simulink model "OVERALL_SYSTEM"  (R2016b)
settings: Solver=VariableStepAuto  StartTime=0.0  StopTime=12  FixedStep=0.1e-3  RelTol=1e-3
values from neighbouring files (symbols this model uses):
  beta_max = 90    [SYSTEM_PATAMETERS.m]
  beta_min = 0    [SYSTEM_PATAMETERS.m]
  beta_r = 4    [SYSTEM_PATAMETERS.m]
  c1 = 0.5    [SYSTEM_PATAMETERS.m]
  c2 = 116    [SYSTEM_PATAMETERS.m]
  c3 = 0.4    [SYSTEM_PATAMETERS.m]
  c4 = 5    [SYSTEM_PATAMETERS.m]
  c5 = 21    [SYSTEM_PATAMETERS.m]
  c6 = 0    [SYSTEM_PATAMETERS.m]
  Cdc = 0.08    [SYSTEM_PATAMETERS.m]
  Cp_max = 0.41    [SYSTEM_PATAMETERS.m]
  fn = 50    [SYSTEM_PATAMETERS.m]
  I2base = (2*Sn)/(3*V2base)    [SYSTEM_PATAMETERS.m]
  Ibase = (2*Sn)/(3*Vbase)    [SYSTEM_PATAMETERS.m]
  Idcbase = ((3/2)*Vbase*Ibase)/Vdcbase    [SYSTEM_PATAMETERS.m]
  J = Sn*2*H/(wm^2)    (= 133997.265367)    [SYSTEM_PATAMETERS.m]
  Ki = Kp/Ti    (= 750)    [SYSTEM_PATAMETERS.m]
  Ki_SSC = Kp_SSC/Ti_SSC    [SYSTEM_PATAMETERS.m]
  Kib = Kpb/Tb    (= 25)    [SYSTEM_PATAMETERS.m]
  Kibv = Kpbv/Tibv    [SYSTEM_PATAMETERS.m]
  Kidc = Kpdc/Tidc    [SYSTEM_PATAMETERS.m]
  Kiq = Kpq/Tiq    [SYSTEM_PATAMETERS.m]
  Kiw = Kpw/Tiw    (= 1)    [SYSTEM_PATAMETERS.m]
  Kp = xs_filter/(2*wbase*Ta)    (= 12.7323954474)    [SYSTEM_PATAMETERS.m]
  Kp_SSC = ls_filter/(2*wbase*Te)    [SYSTEM_PATAMETERS.m]
  Kpb = 5    [SYSTEM_PATAMETERS.m]
  Kpbv = ls_filterb/(2*wbase*Te)    [SYSTEM_PATAMETERS.m]
  Kpdc = (Vdcbase*Tc)/(V2*a*Teq)    [SYSTEM_PATAMETERS.m]
  Kpq = Tf_Q_const*rs_filter/(a*Teq)    [SYSTEM_PATAMETERS.m]
  Kpw = 4    [SYSTEM_PATAMETERS.m]
  lambda_opt = 7.95    [SYSTEM_PATAMETERS.m]
  ls = Ls/Lbase    [SYSTEM_PATAMETERS.m]
  ls_filter = Ls_filter/Lbase    [SYSTEM_PATAMETERS.m]
  Ls_filter = Xs_filter/we    [SYSTEM_PATAMETERS.m]
  polepairs = poles/2    (= 115)    [SYSTEM_PATAMETERS.m]
  psim_pu = psim/psibase    [SYSTEM_PATAMETERS.m]
  r = 26    [SYSTEM_PATAMETERS.m]
  rho = 1.225    [SYSTEM_PATAMETERS.m]
  Rs = rs*Zbase    [SYSTEM_PATAMETERS.m]
  Rs_filter = rs_filter*Zbase    [SYSTEM_PATAMETERS.m]
  Sn = 250e3    (= 250000)    [SYSTEM_PATAMETERS.m]
  Ta = Tsw/2    (= 0.0001)    [SYSTEM_PATAMETERS.m]
  Ts = 1e-5    (= 1e-05)    [SYSTEM_PATAMETERS.m]
  V2 = 400    [SYSTEM_PATAMETERS.m]
  V2base = V2*sqrt(2)/sqrt(3)    [SYSTEM_PATAMETERS.m]
  Vbase = V1*sqrt(2)/sqrt(3)    [SYSTEM_PATAMETERS.m]
  Vdcbase = 3*Vbase    [SYSTEM_PATAMETERS.m]
  w2base = 2*pi*fn    (= 314.159265359)    [SYSTEM_PATAMETERS.m]
  wbase = 2*pi*fn    (= 314.159265359)    [SYSTEM_PATAMETERS.m]
  wm = nm*pi/30    (= 2.73181969877)    [SYSTEM_PATAMETERS.m]
undefined symbols (not defined in the file or in its folder): bridge, by, dend, DiscIntNeverNeededParam, established, Flux, h, Ion, K, Ld, linkage, Lithium, Lq, magnets, numd, phase, Pm0, pulses, sigbuilder_block, Td, Three, Tlim, Tr, V
libraries: powerlib x32, powerlib_meascontrol x14, simulink x10, powerlib_extras x2, sps_avr x1, electricdrivelib x1
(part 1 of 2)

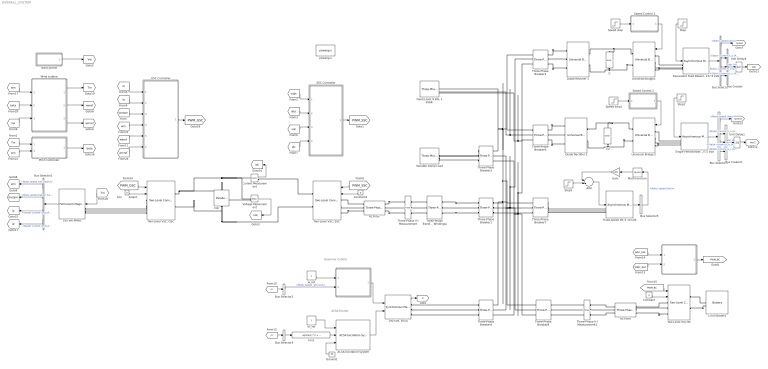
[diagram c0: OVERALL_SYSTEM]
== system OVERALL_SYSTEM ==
  note: Governor Control
  note: AC5A Exciter
  " " : Subsystem
  " " : Subsystem
  "140 kVA, EESG" : powerlib/Machines/Synchronous Machine pu Fundamental  PresetModel=No  MechanicalLoad=Mechanical power Pm  ShowDetailedParameters=on  RotorType=Round  Units=per unit fundamental parameters  MeasurementBus=off  NominalParameters="[ 140e3 V2   fn]"  Stator="[ 0.0317  0.114  1.19  0.36 ]"  Field="[ 5.79E-04  0.114]"  Dampers2=[0.0652, 0.5134, 0.0287, 0.2553, 7.765e-3, 0.9167 ]  Dampers1="[ 1.17E-02  0.182  1.97E-02  0.384 ]"  Mechanical=[ 0.7 0 20]  PolePairs=2  InitialConditions="[ 0  36.87  0  0  0  0  0 0  1 ]"  SetSaturation=off  Saturation=[0.6404,0.7127,0.8441,0.9214,0.9956,1.082,1.19,1.316,1.457;0.7,0.7698,0.8872,0.9466,0.9969,1.046,1.1,1.151,1.201]  LoadFlowParameters=[1,0,0,0,0]  TsPowergui=0  TsBlock=-1  IterativeModel=Trapezoidal non iterative  IterativeDiscreteModel=Trapezoidal non iterative  BusType=PV  Pref=0  Qref=0  Qmin=-inf  Qmax=inf  PLF=0  QLF=0
  250 kW PMSG : powerlib/Machines/Permanent Magnet Synchronous Machine  NbPhases=3  FluxDistribution=Sinusoidal  RotorType=Round  MechanicalLoad=Torque Tm  PresetModel=No  ShowDetailedParameters=on  MeasurementBus=off  Resistance=Rs  Inductance=8.5e-3  dqInductances=[Ld, Lq]  La=Ls  MachineConstant=Flux linkage established by magnets (V.s)  Flux=1.5  VoltageCst=31288.039  TorqueCst=258.75  Flat=120  Mechanical=[J 0 polepairs 0]  PolePairs=273  InitialConditions=[1.76,15, 0,0]  InitialConditions5ph=[0 0 0 0 0 0]  TsPowergui=0  TsBlock=Ts  RefAngle=Aligned with phase A axis (original Park)
  AC5A Excitation System : sps_avr/AC5A Excitation System  Tr=20e-3  KaTa=[500 0.02]  VRminmax=[-7.3 7.3]  KfTf=[0.03 1 0 0]  KeTe=[1 0.02]  Efd12=[5.6 0.75*5.6]  SeEfd12=[0.86 0.5]  v0=[1 1]  TsBlock=0
  Add : Sum
  Bus Creator : BusCreator  Inputs=3
  Bus Creator1 : BusCreator  Inputs=3
  Bus Selector : BusSelector  OutputSignals=Mechanical.Rotor speed (wm),Stator measurements.Stator current is_a (A),Stator measurements.Stator current is_b (A),Stator measurements.Stator current is_c (A)
  Bus Selector1 : BusSelector  OutputSignals=Rotor speed wm (rad/s),Rotor angle thetam (rad),Stator current is_q (A),Stator current is_d (A)
  Bus Selector2 : BusSelector  OutputSignals="Mechanical.Rotor speed  wm (pu)"
  Bus Selector3 : BusSelector  OutputSignals="dq0 components.Stator voltage  vq (pu),dq0 components.Stator voltage  vd (pu)"  OutputAsBus=on
  Bus Selector4 : BusSelector  OutputSignals=Mechanical.Rotor speed (wm),Stator measurements.Stator current is_a (A),Stator measurements.Stator current is_b (A),Stator measurements.Stator current is_c (A)
  Bus Selector5 : BusSelector  OutputSignals=Mechanical.Rotor speed (wm)
  C : powerlib/Elements/Series RLC Branch  LConnTagsString=__new0  RConnTagsString=__new0  BranchType=C  Resistance=1  Inductance=1e-3  SetiL0=off  InitialCurrent=0  Capacitance=7.5e-3  Setx0=on  InitialVoltage=sqrt(2)*400  Measurements=None
  C2 : powerlib/Elements/Series RLC Branch  LConnTagsString=__new0  RConnTagsString=__new0  BranchType=C  Resistance=1  Inductance=1e-3  SetiL0=off  InitialCurrent=0  Capacitance=7.5e-3  Setx0=on  InitialVoltage=sqrt(2)*400  Measurements=None
  Cdc : powerlib/Elements/Parallel RLC Branch  LConnTagsString=a  RConnTagsString=__new0  BranchType=C  Resistance=1e12  Inductance=1e-3  SetiL0=off  InitialCurrent=0  Capacitance=Cdc  Setx0=on  InitialVoltage=Vdcbase  Measurements=None
  Con        2stant : Constant  Value=0
  Constant : Constant  Value=0
  Constant1 : Constant  Value=0
  Current Measurement : powerlib/Measurements/Current Measurement  PhasorSimulation=off  OutputType=Complex  PSBequivalent=0
  Diode Rectifier 1 : powerlib/Power Electronics/Universal Bridge  Arms=3  SnubberResistance=1e5  SnubberCapacitance=inf  Device=Diodes  Ron=1e-3  Lon=0  ForwardVoltages="[  0  0  ]"  ForwardVoltage=0  GTOparameters=[ 10e-6 , 20e-6 ]  IGBTparameters=[ 1e-6 , 2e-6 ]  Measurements=None  Measurements_2=None  converterType=Rectifier
  Diode Rectifier 2 : powerlib/Power Electronics/Universal Bridge  Arms=3  SnubberResistance=1e5  SnubberCapacitance=inf  Device=Diodes  Ron=1e-3  Lon=0  ForwardVoltages="[  0  0  ]"  ForwardVoltage=0  GTOparameters=[ 10e-6 , 20e-6 ]  IGBTparameters=[ 1e-6 , 2e-6 ]  Measurements=None  Measurements_2=None  converterType=Rectifier
  "Equivalent Feed Blower, 137.5 kVA" : powerlib/Machines/Asynchronous Machine SI Units  RotorType=Squirrel-cage  PresetModel=No  MechanicalLoad=Torque Tm  ShowDetailedParameters=on  ReferenceFrame=Stationary  Units=SI  MeasurementBus=off  NominalParameters=[137.5e3 400 50]  Stator=[ 0.087 0.8e-3 ]  Rotor="[ 0.228  0.8e-3 ]"  Cage1=[0.4155 0.002066]  Cage2=[0.4168 0.0003495]  Lm=0.0354  Mechanical="[1.662  0.01 2 ]"  PolePairs=2  InitialConditions=[1 0 0 0 0 0 0 0]  SimulateSaturation=off  Saturation=[14.03593122, 27.81365428, 53.79336849, 72.68890987, 97.98006896, 148.6815601, 215.7428561, 302.9841135, 428.7778367 ; 230, 322, 414, 460, 506, 552, 598, 644, 690]  LoadFlowParameters=1492000  TsPowergui=0  TsBlock=-1  IterativeModel=Trapezoidal non iterative  IterativeDiscreteModel=Trapezoidal non iterative  Pmec=72.6e3
  Fcn1 : Fcn  Expr=sqrt(u(1)^2 + u(2)^2)
  "Fixed Load, 9 kW, 1 kVAR " : powerlib/Elements/Three-Phase Series RLC Load  LConnTagsString=A|B|C  Configuration=Y (grounded)  NominalVoltage=400  Vabc=[1e3 1e3 1e3]  Vabcp=[1e3 1e3 1e3]  NominalFrequency=50  UnbalancedPower=off  ActivePower=2e3  InductivePower=0.5e3  CapacitivePower=0  Pabc=[10e3 9e3 11e3]  QLabc=[100 90 110]  QCabc=[100 90 110]  Pabcp=[10e3 9e3 11e3]  QLabcp=[100 90 110]  QCabcp=[100 90 110]  Measurements=None  LoadType=constant Z
  "Fixed-speed IM, 5-10 kVA" : powerlib/Machines/Asynchronous Machine pu Units  RotorType=Squirrel-cage  PresetModel=No  MechanicalLoad=Torque Tm  ShowDetailedParameters=on  ReferenceFrame=Rotor  Units=pu  MeasurementBus=off  NominalParameters=[10000 400 50]  Stator=[0.01965 0.0397]  Rotor=[0.01909 0.0397]  Cage1=[0.01909 0.0397]  Cage2=[0.01909 0.0397]  Lm=1.354  Mechanical=[0.6 0.05479 2]  PolePairs=2  InitialConditions="[ 1,0   0,0,0   0,0,0 ]"  SimulateSaturation=off  Saturation="[0.212,0.4201,0.8125,1.0979,1.4799,2.2457,3.2586,4.5763,6.4763 ;   0.5,0.7,0.9,1,1.1,1.2 ,1.3,1.4,1.5]"  LoadFlowParameters=0  TsPowergui=0  TsBlock=-1  IterativeModel=Trapezoidal non iterative  IterativeDiscreteModel=Trapezoidal non iterative  Pmec=0
  GSC Controller : Subsystem
  Gain : Gain  Gain=0.85
  Ground1 : Ground
  Li-ion Battery : electricdrivelib/Extra Sources/Battery  BatType=Lithium-Ion  ShowTempParam=off  ThermalPreset=no  NomV=Vb  NomQ=Ahb  SOC=SOC0  Batt_Tr=0.1  PresetModel=on  MaxQ=100  MinV=739.5  FullV=1147.6913  Dis_rate=43.4783  R=0.0986  Normal_OP=90.4348  expZone="[1065.2605      4.9130435]"  current=[50]  Units=Ampere-hour  Tci=20  NomT=25  T2=0  MaxQ2=2.208  FullV2=3.45  Normal_OP2=2.8  expZone2="[3.22        0.23]"  Rca=0.6  ti=1000  Dp=0
  Math Function : Math  Operator=square
  Pitch Controller : Subsystem
  RL Filter : powerlib/Elements/Three-Phase Series RLC Branch  LConnTagsString=A|B|C  RConnTagsString=A|B|C  BranchType=RL  Resistance=Rs_filter  Inductance=Ls_filter  Capacitance=1e-6  Measurements=None
  RL-Filter : powerlib/Elements/Three-Phase Series RLC Branch  LConnTagsString=A|B|C  RConnTagsString=A|B|C  BranchType=RL  Resistance=Rs_filter  Inductance=Ls_filter  Capacitance=1e-6  Measurements=None
  SSC Controller : Subsystem
  "Single Feed Blower, 27.5 kVA" : powerlib/Machines/Asynchronous Machine SI Units  RotorType=Squirrel-cage  PresetModel=No  MechanicalLoad=Torque Tm  ShowDetailedParameters=on  ReferenceFrame=Stationary  Units=SI  MeasurementBus=off  NominalParameters=[27.5e3 400 50]  Stator=[ 0.087 0.8e-3 ]  Rotor="[ 0.228  0.8e-3 ]"  Cage1=[0.4155 0.002066]  Cage2=[0.4168 0.0003495]  Lm=0.0354  Mechanical="[1.662  0.01 2 ]"  PolePairs=2  InitialConditions=[1 0 0 0 0 0 0 0]  SimulateSaturation=off  Saturation=[14.03593122, 27.81365428, 53.79336849, 72.68890987, 97.98006896, 148.6815601, 215.7428561, 302.9841135, 428.7778367 ; 230, 322, 414, 460, 506, 552, 598, 644, 690]  LoadFlowParameters=1492000  TsPowergui=0  TsBlock=-1  IterativeModel=Trapezoidal non iterative  IterativeDiscreteModel=Trapezoidal non iterative  Pmec=72.6e3
  Speed step : Step  Time=3  After=150  SampleTime=0
  Speed step1 : Step  Time=3  After=150  SampleTime=0
  Speed Control 1 : Subsystem
  Speed Control 2 : Subsystem
  Step : Step  Time=4  After=240  SampleTime=0
  Step1 : Step  Time=4  After=150  SampleTime=0
  Step2 : Step  Time=6  After=0.15  SampleTime=0
  Three-Phase Transformer (Two Windings) : powerlib/Elements/Three-Phase Transformer (Two Windings)  Winding1Connection=Yg  Winding2Connection=Yg  CoreType=Three single-phase transformers  SetSaturation=off  Hysteresis=off  DataFile='hysteresis'  SetInitialFlux=off  Measurements=None  UNITS=pu  NominalPower=[ 250e3 , 50 ]  Winding1=[ 690 , 0.002 , 0.08 ]  Winding2=[ 400 , 0.002 , 0.08 ]  Rm=500  Lm=500  L0=0.5  Saturation=[ 0,0 ; 0.0024,1.2 ; 1.0,1.52 ]  InitialFluxes=[ 0.8 , -0.8 , 0.7 ]  MoreParameters=off  BreakLoop=off  DataType=off  TransfoNumber=1
  Three-Phase V-I Measurement : powerlib/Measurements/Three-Phase V-I Measurement  VoltageMeasurement=phase-to-phase  SetLabelV=on  LabelV=vabc  Vpu=off  VpuLL=off  CurrentMeasurement=yes  SetLabelI=on  LabelI=iabc  Ipu=off  Pbase=6e6  Vbase=690  OutputType=Complex  PhasorSimulation=off  PSBequivalent=0
  Three-Phase V-I Measurement1 : powerlib/Measurements/Three-Phase V-I Measurement  VoltageMeasurement=phase-to-phase  SetLabelV=on  LabelV=Vabc_bat  Vpu=off  VpuLL=off  CurrentMeasurement=yes  SetLabelI=on  LabelI=Iabc_bat  Ipu=off  Pbase=6e6  Vbase=690  OutputType=Complex  PhasorSimulation=off  PSBequivalent=0
  Three-Phase Breaker{1..3,6} (4 alike) : powerlib/Elements/Three-Phase Breaker  InitialState=open  SwitchA=on  SwitchB=on  SwitchC=on  SwitchTimes=2.9  External=off  BreakerResistance=0.01  SnubberResistance=1e6  SnubberCapacitance=inf  Measurements=None
  Three-Phase Breaker4 : powerlib/Elements/Three-Phase Breaker  InitialState=open  SwitchA=on  SwitchB=on  SwitchC=on  SwitchTimes=5.25  External=off  BreakerResistance=0.01  SnubberResistance=1e6  SnubberCapacitance=inf  Measurements=None
  Three-Phase Breaker7 : powerlib/Elements/Three-Phase Breaker  InitialState=open  SwitchA=on  SwitchB=on  SwitchC=on  SwitchTimes=6  External=off  BreakerResistance=0.01  SnubberResistance=1e6  SnubberCapacitance=inf  Measurements=None
  Three-Phase Breaker8 : powerlib/Elements/Three-Phase Breaker  InitialState=open  SwitchA=on  SwitchB=on  SwitchC=on  SwitchTimes=5.25  External=off  BreakerResistance=0.01  SnubberResistance=1e6  SnubberCapacitance=inf  Measurements=None
  Two-Level VSC BC : powerlib/Power Electronics/Two-Level Converter  ModelType=Switching devices  Ron=1e-3  Rs=1e6  Cs=inf  Vforward=[0,0]  Ron_Diode=1e-3  Rs_Diode=1e6  Cs_Diode=inf  Vf_Diode=1e-3  Rs_CurrentSource=inf
  "Two-Level VSC, GSC" : powerlib/Power Electronics/Two-Level Converter  ModelType=Switching devices  Ron=1e-3  Rs=1e6  Cs=inf  Vforward=[0,0]  Ron_Diode=1e-3  Rs_Diode=1e6  Cs_Diode=inf  Vf_Diode=1e-3  Rs_CurrentSource=inf
  "Two-Level VSC, SSC" : powerlib/Power Electronics/Two-Level Converter  ModelType=Switching devices  Ron=1e-3  Rs=1e6  Cs=inf  Vforward=[0,0]  Ron_Diode=1e-3  Rs_Diode=1e6  Cs_Diode=inf  Vf_Diode=1e-3  Rs_CurrentSource=inf
  Unit Delay1 : UnitDelay  SampleTime=Ts
  Unit Delay4 : UnitDelay  SampleTime=Ts
  Universal Bridge 2 : powerlib/Power Electronics/Universal Bridge  Arms=3  SnubberResistance=1e5  SnubberCapacitance=inf  Device=IGBT / Diodes  Ron=1e-3  Lon=0  ForwardVoltages="[  0  0  ]"  ForwardVoltage=0  GTOparameters=[ 10e-6 , 20e-6 ]  IGBTparameters=[ 1e-6 , 2e-6 ]  Measurements=None  Measurements_2=None  converterType=Rectifier
  Universal Bridge1 : powerlib/Power Electronics/Universal Bridge  Arms=3  SnubberResistance=1e5  SnubberCapacitance=inf  Device=IGBT / Diodes  Ron=1e-3  Lon=0  ForwardVoltages="[  0  0  ]"  ForwardVoltage=0  GTOparameters=[ 10e-6 , 20e-6 ]  IGBTparameters=[ 1e-6 , 2e-6 ]  Measurements=None  Measurements_2=None  converterType=Rectifier
  Variable Dump Load : powerlib/Elements/Three-Phase Series RLC Load  LConnTagsString=A|B|C  Configuration=Y (grounded)  NominalVoltage=400  Vabc=[1e3 1e3 1e3]  Vabcp=[1e3 1e3 1e3]  NominalFrequency=50  UnbalancedPower=off  ActivePower=10e3  InductivePower=1e3  CapacitivePower=0  Pabc=[10e3 9e3 11e3]  QLabc=[100 90 110]  QCabc=[100 90 110]  Pabcp=[10e3 9e3 11e3]  QLabcp=[100 90 110]  QCabcp=[100 90 110]  Measurements=None  LoadType=constant Z
  Voltage Measurement : powerlib/Measurements/Voltage Measurement  PhasorSimulation=off  OutputType=Complex  PSBequivalent=0
  Vt_ref : Constant
  Wind profile : Subsystem  Tag=STV Subsys  LoadFcn=sigbuilder_block('load');  StartFcn=sigbuilder_block('start');  StopFcn=sigbuilder_block('stop');  ClipboardFcn=sigbuilder_block('clipboard');
  Wind turbine : Subsystem
  powergui : powerlib/powergui  Priority=1  SimulationMode=Discrete  SolverType=Tustin/Backward Euler (TBE)  SampleTime=Ts  frequency=60  SPID=off  DisableSnubberDevices=off  DisableRonSwitches=off  DisableVfSwitches=off  SwTol=0  DisplayEquations=off  Interpol=off  ExternalGateDelay=off  methode=off  Ts=10  FunctionMessages=off  echomessages=off  HookPort=off  EnableUseOfTLC=off  x0status=blocks  frequencyindice=50  Pbase=100e6  ErrMax=1e-4  Iterations=50  UnitsV=kV  UnitsW=MW  buscounter=0  RestoreLinks=warning  ResistiveCurrentMeasurement=off  Frange=[0:2:500]  Ylog=off  Xlog=on  ShowGrid=off  save=off  variable=ZData  structure=0  ZoomFFT=off  StartTime=0.0  cycles=1  DisplayStyle=1  fundamental=60  FreqAxis=off  MaxFrequency=1000  frequencyindicesteady=1  RmsSteady=1  display=off
  w_ref : Constant
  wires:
  Bus Selector1/2 -> [thetam]  "<Rotor angle thetam (rad)>"
  Bus Selector1/1 -> [wm]  "<Rotor speed wm (rad/s)>"
  Bus Selector1/3 -> [iq]  "<Stator current is_q (A)>"
  Bus Selector1/4 -> [id]  "<Stator current is_d (A)>"
  Con        2stant/1 -> "Two-Level VSC, GSC"/2
  [Tm] -> 250 kW PMSG/1
  [beta] -> Wind turbine/2(Beta [deg])
  [wm] -> Wind turbine/1("wm [rad/s] ")
  Wind turbine/1(Tm [Nm]) -> [Tm]
  Wind turbine/2(we_ref [pu]) -> [weref]
  [PWM_GSC] -> "Two-Level VSC, GSC"/1
  GSC Controller/1(Uref) -> [PWM_GSC]
  [id] -> GSC Controller/1(Id [A])
  [iq] -> GSC Controller/2(Iq [A])
  [thetam] -> GSC Controller/3(Thetam [rad])
  [wm] -> GSC Controller/4(Wm [rad/s])
  [weref] -> GSC Controller/5(We_ref [pu])
  Constant1/1 -> "Two-Level VSC, SSC"/2
  [PWM_SSC] -> "Two-Level VSC, SSC"/1
  Voltage Measurement/1 -> [vdc]
  Current Measurement/1 -> [idc]
  SSC Controller/1(Uref) -> [PWM_SSC]
  [vabc] -> SSC Controller/1(vabc [V])
  [iabc] -> SSC Controller/2(iabc [A])
  [vdc] -> SSC Controller/3(vdc [V])
  [idc] -> SSC Controller/4(idc [A])
  [Tm] -> Pitch Controller/1(Tm [Nm])
  Pitch Controller/1(Beta [deg]) -> [beta]
  [Vw] -> Wind turbine/3(V_wind [m/s])
  [wm] -> Pitch Controller/2(wm [rad/s])
  Wind turbine/3(wm_ref [pu]) -> [wmref]
  [wmref] -> GSC Controller/6(Wm_ref [pu])
  250 kW PMSG/1 -> Bus Selector1/1
  Wind profile/1(Final Wind) -> [Vw]
  Ground1/1 -> AC5A Excitation System/3
  AC5A Excitation System/1 -> "140 kVA, EESG"/2
  Vt_ref/1 -> AC5A Excitation System/1
  Fcn1/1 -> AC5A Excitation System/2
  Bus Selector3/1 -> Fcn1/1
  Bus Selector2/1 -> " "/2(w (pu))  "<Rotor speed  wm (pu)>"
  w_ref/1 -> " "/1(wref (pu))
  " "/1(Pmec (pu)) -> "140 kVA, EESG"/1
  "140 kVA, EESG"/1 -> [m]
  [m] -> Bus Selector2/1
  [m] -> Bus Selector3/1
  Constant/1 -> Two-Level VSC BC/2
  " "/1(Vref) -> [PWM_BC]
  [Vabc_bat] -> " "/2(Vabc [V])
  [Iabc_bat] -> " "/1(Iabc [A])
  [PWM_BC] -> Two-Level VSC BC/1
  Unit Delay4/1 -> [Iabc]
  Bus Selector/3 -> Bus Creator/2  "<Stator current is_b (A)>"
  Bus Creator/1 -> Unit Delay4/1  "Iabc (A)"
  Bus Selector/2 -> Bus Creator/1  "<Stator current is_a (A)>"
  Bus Selector/4 -> Bus Creator/3  "<Stator current is_c (A)>"
  Speed Control 1/1(pulses) -> Universal Bridge1/1
  Step/1 -> "Equivalent Feed Blower, 137.5 kVA"/1
  Speed step/1 -> Speed Control 1/1(speed)
  "Equivalent Feed Blower, 137.5 kVA"/1 -> Bus Selector/1
  Bus Selector/1 -> [Speed]  "<Rotor speed (wm)>"
  Speed Control 2/1(pulses) -> Universal Bridge 2/1
  Step1/1 -> "Single Feed Blower, 27.5 kVA"/1
  Speed step1/1 -> Speed Control 2/1(speed)
  Unit Delay1/1 -> [Iabc2]
  Bus Selector4/3 -> Bus Creator1/2  "<Stator current is_b (A)>"
  Bus Creator1/1 -> Unit Delay1/1  "Iabc (A)"
  Bus Selector4/2 -> Bus Creator1/1  "<Stator current is_a (A)>"
  Bus Selector4/4 -> Bus Creator1/3  "<Stator current is_c (A)>"
  "Single Feed Blower, 27.5 kVA"/1 -> Bus Selector4/1
  Bus Selector4/1 -> [Speed2]  "<Rotor speed (wm)>"
  Step2/1 -> Add/2
  "Fixed-speed IM, 5-10 kVA"/1 -> Bus Selector5/1
  Bus Selector5/1 -> Math Function/1  "<Rotor speed (wm)>"
  Add/1 -> "Fixed-speed IM, 5-10 kVA"/1
  Math Function/1 -> Gain/1
  Gain/1 -> Add/1
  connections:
  Three-Phase Breaker3/RConn1 -- Variable Dump Load/LConn1
  Variable Dump Load/LConn2 -- Three-Phase Breaker3/RConn2
  Three-Phase Breaker3/RConn3 -- Variable Dump Load/LConn3
  "140 kVA, EESG"/RConn1 -- Three-Phase Breaker4/LConn1
  "140 kVA, EESG"/RConn2 -- Three-Phase Breaker4/LConn2
  "140 kVA, EESG"/RConn3 -- Three-Phase Breaker4/LConn3
  Cdc/RConn1 -- "Two-Level VSC, SSC"/RConn2 -- Voltage Measurement/LConn2 -- "Two-Level VSC, GSC"/RConn2
  "Two-Level VSC, GSC"/RConn1 -- Current Measurement/LConn1 -- Voltage Measurement/LConn1 -- Cdc/LConn1
  "Two-Level VSC, SSC"/RConn1 -- Current Measurement/RConn1
  RL Filter/LConn3 -- Three-Phase V-I Measurement/RConn3
  "Two-Level VSC, SSC"/LConn1 -- RL Filter/RConn1
  "Two-Level VSC, GSC"/LConn3 -- 250 kW PMSG/LConn3
  "Two-Level VSC, GSC"/LConn1 -- 250 kW PMSG/LConn1
  "Two-Level VSC, SSC"/LConn2 -- RL Filter/RConn2
  "Two-Level VSC, GSC"/LConn2 -- 250 kW PMSG/LConn2
  RL Filter/LConn1 -- Three-Phase V-I Measurement/RConn1
  "Two-Level VSC, SSC"/LConn3 -- RL Filter/RConn3
  RL Filter/LConn2 -- Three-Phase V-I Measurement/RConn2
  RL-Filter/RConn1 -- Two-Level VSC BC/LConn1
  RL-Filter/RConn2 -- Two-Level VSC BC/LConn2
  RL-Filter/RConn3 -- Two-Level VSC BC/LConn3
  Li-ion Battery/LConn2 -- Two-Level VSC BC/RConn2
  Li-ion Battery/LConn1 -- Two-Level VSC BC/RConn1
  Three-Phase V-I Measurement/LConn1 -- Three-Phase Transformer (Two Windings)/LConn1
  Three-Phase V-I Measurement/LConn2 -- Three-Phase Transformer (Two Windings)/LConn2
  Three-Phase V-I Measurement/LConn3 -- Three-Phase Transformer (Two Windings)/LConn3
  Three-Phase Breaker1/LConn2 -- Three-Phase Transformer (Two Windings)/RConn2
  Three-Phase Transformer (Two Windings)/RConn1 -- Three-Phase Breaker1/LConn1
  Three-Phase Transformer (Two Windings)/RConn3 -- Three-Phase Breaker1/LConn3
  Universal Bridge1/RConn1 -- Diode Rectifier 1/RConn1 -- C/LConn1
  C/RConn1 -- Universal Bridge1/RConn2 -- Diode Rectifier 1/RConn2
  Universal Bridge1/LConn1 -- "Equivalent Feed Blower, 137.5 kVA"/LConn1
  Universal Bridge1/LConn2 -- "Equivalent Feed Blower, 137.5 kVA"/LConn2
  Universal Bridge1/LConn3 -- "Equivalent Feed Blower, 137.5 kVA"/LConn3
  Universal Bridge 2/RConn1 -- C2/LConn1 -- Diode Rectifier 2/RConn1
  C2/RConn1 -- Universal Bridge 2/RConn2 -- Diode Rectifier 2/RConn2
  Universal Bridge 2/LConn1 -- "Single Feed Blower, 27.5 kVA"/LConn1
  Universal Bridge 2/LConn2 -- "Single Feed Blower, 27.5 kVA"/LConn2
  Universal Bridge 2/LConn3 -- "Single Feed Blower, 27.5 kVA"/LConn3
  Three-Phase Breaker7/RConn1 -- "Fixed-speed IM, 5-10 kVA"/LConn1
  Three-Phase Breaker7/RConn2 -- "Fixed-speed IM, 5-10 kVA"/LConn2
  Three-Phase Breaker7/RConn3 -- "Fixed-speed IM, 5-10 kVA"/LConn3
  Three-Phase Breaker2/RConn2 -- Diode Rectifier 1/LConn2
  Three-Phase Breaker2/RConn1 -- Diode Rectifier 1/LConn1
  Three-Phase Breaker2/RConn3 -- Diode Rectifier 1/LConn3
  Three-Phase Breaker6/RConn2 -- Diode Rectifier 2/LConn2
  Three-Phase Breaker6/RConn1 -- Diode Rectifier 2/LConn1
  Three-Phase Breaker6/RConn3 -- Diode Rectifier 2/LConn3
  Three-Phase V-I Measurement1/RConn1 -- Three-Phase Breaker8/RConn1
  Three-Phase V-I Measurement1/RConn2 -- Three-Phase Breaker8/RConn2
  Three-Phase V-I Measurement1/RConn3 -- Three-Phase Breaker8/RConn3
  Three-Phase V-I Measurement1/LConn2 -- RL-Filter/LConn2
  Three-Phase V-I Measurement1/LConn1 -- RL-Filter/LConn1
  Three-Phase V-I Measurement1/LConn3 -- RL-Filter/LConn3
  Three-Phase Breaker6/LConn1 -- Three-Phase Breaker2/LConn1 -- "Fixed Load, 9 kW, 1 kVAR "/LConn1 -- Three-Phase Breaker3/LConn1 -- Three-Phase Breaker8/LConn1 -- Three-Phase Breaker4/RConn1 -- Three-Phase Breaker7/LConn1 -- Three-Phase Breaker1/RConn1
  Three-Phase Breaker1/RConn2 -- Three-Phase Breaker4/RConn2 -- Three-Phase Breaker8/LConn2 -- Three-Phase Breaker2/LConn2 -- "Fixed Load, 9 kW, 1 kVAR "/LConn2 -- Three-Phase Breaker6/LConn2 -- Three-Phase Breaker3/LConn2 -- Three-Phase Breaker7/LConn2
  Three-Phase Breaker1/RConn3 -- Three-Phase Breaker8/LConn3 -- Three-Phase Breaker4/RConn3 -- Three-Phase Breaker2/LConn3 -- "Fixed Load, 9 kW, 1 kVAR "/LConn3 -- Three-Phase Breaker6/LConn3 -- Three-Phase Breaker3/LConn3 -- Three-Phase Breaker7/LConn3

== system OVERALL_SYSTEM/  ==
  note: Actuator
  note: Controller
  wref (pu) : Inport
  w (pu) : Inport  Port=2
  Gain Kpc : Gain  Gain=K
  Integrator : Integrator  InitialCondition=Pm0  LimitOutput=on  UpperSaturationLimit=Tlim(2)  LowerSaturationLimit=Tlim(1)
  Product : Product
  Sum : Sum  Inputs=+-
  TF : TransferFcn  Numerator=([Tr(3) 1])  Denominator="([Tr(1)*Tr(2)  Tr(1) 1])"
  TF1 : TransferFcn  Numerator=([Ta(1) 1])  Denominator=([Ta(2) 1])
  TF2 : TransferFcn  Numerator=1  Denominator=([Ta(3) 1])
  Time-Delay : TransportDelay  DelayTime=Td  InitialOutput=Pm0
  Pmec (pu) : Outport  InitialOutput=0
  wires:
  Integrator/1 -> Time-Delay/1  "Torque"
  TF2/1 -> Integrator/1
  Product/1 -> Pmec (pu)/1
  wref (pu)/1 -> Sum/1
  Time-Delay/1 -> Product/1
  w (pu)/1 -> Sum/2, Product/2
  TF1/1 -> TF2/1
  TF/1 -> Gain Kpc/1
  Sum/1 -> TF/1
  Gain Kpc/1 -> TF1/1

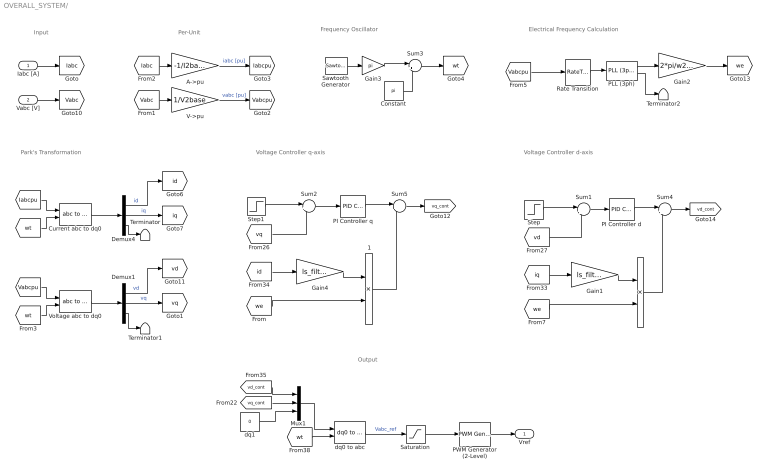
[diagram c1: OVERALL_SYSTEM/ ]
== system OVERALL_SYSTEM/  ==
  note: Input
  note: Voltage Controller d-axis
  note: Per-Unit
  note: Voltage Controller q-axis
  note: Park's Transformation
  note: Electrical Frequency Calculation
  note: Frequency Oscillator
  note: Output
  Iabc [A] : Inport
  Vabc [V] : Inport  Port=2
  " 1" : Product
  A->pu : Gain  Gain=-1/I2base
  Constant : Constant  Value=pi
  Current abc to dq0 : powerlib_meascontrol/Transformations/abc to dq0  Alignment=90 degrees behind phase A axis
  Demux1 : Demux  Outputs=3
  Demux4 : Demux  Outputs=3
  Gain1 : Gain  Gain=ls_filter
  Gain2 : Gain  Gain=2*pi/w2base
  Gain3 : Gain  Gain=pi
  Gain4 : Gain  Gain=ls_filter
  Mux1 : Mux  Inputs=3
  PI Controller d : simulink/Continuous/PID Controller  Controller=PI  TimeDomain=Continuous-time  SampleTime=-1  IntegratorMethod=Forward Euler  FilterMethod=Forward Euler  Form=Parallel  UseFilter=on  ControllerParametersSource=internal  P=Kpbv  I=Kibv  D=0  N=100  InitialConditionSource=internal  InitialConditionForIntegrator=0  InitialConditionForFilter=0  ExternalReset=none  LimitOutput=off  UpperSaturationLimit=inf  LowerSaturationLimit=-inf  LinearizeAsGain=on  AntiWindupMode=none  Kb=1  TrackingMode=off  Kt=1  PParamMin=[]  PParamMax=[]  IParamMin=[]  IParamMax=[]  DParamMin=[]  DParamMax=[]  NParamMin=[]  NParamMax=[]  KbParamMin=[]  KbParamMax=[]  KtParamMin=[]  KtParamMax=[]  POutMin=[]  POutMax=[]  IOutMin=[]  IOutMax=[]  DOutMin=[]  DOutMax=[]  NOutMin=[]  NOutMax=[]  KbOutMin=[]  KbOutMax=[]  KtOutMin=[]  KtOutMax=[]  IntegratorOutMin=[]  IntegratorOutMax=[]  FilterOutMin=[]  FilterOutMax=[]  SumOutMin=[]  SumOutMax=[]  SumI1OutMin=[]  SumI1OutMax=[]  SumI2OutMin=[]  SumI2OutMax=[]  SumI3OutMin=[]  SumI3OutMax=[]  SumDOutMin=[]  SumDOutMax=[]  SaturationOutMin=[]  SaturationOutMax=[]  IntegratorContinuousStateAttributes=''  IntegratorStateMustResolveToSignalObject=off  IntegratorRTWStateStorageClass=Auto  FilterContinuousStateAttributes=''  FilterStateMustResolveToSignalObject=off  FilterRTWStateStorageClass=Auto  DifferentiatorICPrevScaledInput=0  DifferentiatorOutMin=[]  DifferentiatorOutMax=[]
  PI Controller q : simulink/Continuous/PID Controller  Controller=PI  TimeDomain=Continuous-time  SampleTime=-1  IntegratorMethod=Forward Euler  FilterMethod=Forward Euler  Form=Parallel  UseFilter=on  ControllerParametersSource=internal  P=Kpbv  I=Kibv  D=0  N=100  InitialConditionSource=internal  InitialConditionForIntegrator=0  InitialConditionForFilter=0  ExternalReset=none  LimitOutput=off  UpperSaturationLimit=inf  LowerSaturationLimit=-inf  LinearizeAsGain=on  AntiWindupMode=none  Kb=1  TrackingMode=off  Kt=1  PParamMin=[]  PParamMax=[]  IParamMin=[]  IParamMax=[]  DParamMin=[]  DParamMax=[]  NParamMin=[]  NParamMax=[]  KbParamMin=[]  KbParamMax=[]  KtParamMin=[]  KtParamMax=[]  POutMin=[]  POutMax=[]  IOutMin=[]  IOutMax=[]  DOutMin=[]  DOutMax=[]  NOutMin=[]  NOutMax=[]  KbOutMin=[]  KbOutMax=[]  KtOutMin=[]  KtOutMax=[]  IntegratorOutMin=[]  IntegratorOutMax=[]  FilterOutMin=[]  FilterOutMax=[]  SumOutMin=[]  SumOutMax=[]  SumI1OutMin=[]  SumI1OutMax=[]  SumI2OutMin=[]  SumI2OutMax=[]  SumI3OutMin=[]  SumI3OutMax=[]  SumDOutMin=[]  SumDOutMax=[]  SaturationOutMin=[]  SaturationOutMax=[]  IntegratorContinuousStateAttributes=''  IntegratorStateMustResolveToSignalObject=off  IntegratorRTWStateStorageClass=Auto  FilterContinuousStateAttributes=''  FilterStateMustResolveToSignalObject=off  FilterRTWStateStorageClass=Auto  DifferentiatorICPrevScaledInput=0  DifferentiatorOutMin=[]  DifferentiatorOutMax=[]
  PLL (3ph) : powerlib_meascontrol/PLL/PLL (3ph)  Fmin=1  Par_Init=[0, 50]  ParK=[180, 3200, 1]  TcD=1e-4  MaxRateChangeFreq=12  FilterCutOffFreq=25  Ts=0  AGC=on
  PWM Generator (2-Level) : powerlib_meascontrol/Pulse & Signal Generators/PWM Generator (2-Level)  ModulatorType=Three-phase bridge (6 pulses)  ModulatorMode=Unsynchronized  Fc=fsw  Pc=90  nF=27  MinMax="[ -1  1 ]"  SamplingTechnique=Natural  ModulatingSignals=off  m=0.8  Freq=60  Phase=0  Ts=0  ShowCarrierOutport=off
  Rate Transition : RateTransition  OutPortSampleTime=Ts
  Saturation : Saturate  UpperLimit=10000  LowerLimit=-10000
  Sawtooth Generator : powerlib_meascontrol/Pulse & Signal Generators/Sawtooth Generator  Freq=50  Phase=0  Ts=0
  Step : Step  Time=0  Before=1.732  After=1.732  SampleTime=0
  Step1 : Step  Time=0  After=0  SampleTime=0
  Sum1 : Sum  Inputs=|+-
  Sum2 : Sum  Inputs=|+-
  Sum3 : Sum  Inputs=|++
  Sum4 : Sum  Inputs=|++
  Sum5 : Sum  Inputs=|+-
  Terminator : Terminator
  Terminator1 : Terminator
  Terminator2 : Terminator
  V->pu : Gain  Gain=1/V2base
  Voltage abc to dq0 : powerlib_meascontrol/Transformations/abc to dq0  Alignment=90 degrees behind phase A axis
  dq0 to abc : powerlib_meascontrol/Transformations/dq0 to abc  Alignment=90 degrees behind phase A axis
  dq1 : Constant  Value=0
  Vref : Outport
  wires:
  [iq] -> Gain1/1
  " "/1 -> Sum4/2
  Sum2/1 -> PI Controller q/1
  Gain4/1 -> " 1"/1
  Sum5/1 -> [vq_cont]
  [id] -> Gain4/1
  [Iabc] -> A->pu/1
  [Vabc] -> V->pu/1
  V->pu/1 -> [Vabcpu]  "vabc [pu]"
  A->pu/1 -> [Iabcpu]  "iabc [pu]"
  Sum1/1 -> PI Controller d/1
  Sum4/1 -> [vd_cont]
  Step1/1 -> Sum2/1
  Gain1/1 -> " "/1
  Step/1 -> Sum1/1
  " 1"/1 -> Sum5/2
  Iabc [A]/1 -> [Iabc]
  Vabc [V]/1 -> [Vabc]
  Saturation/1 -> PWM Generator (2-Level)/1
  [wt] -> Voltage abc to dq0/2
  Demux1/3 -> Terminator1/1
  Demux4/1 -> [id]  "id"
  Demux4/3 -> Terminator/1
  [Vabcpu] -> Voltage abc to dq0/1
  Demux4/2 -> [iq]  "iq"
  Current abc to dq0/1 -> Demux4/1
  Voltage abc to dq0/1 -> Demux1/1
  Demux1/1 -> [vd]  "vd"
  [Iabcpu] -> Current abc to dq0/1
  Demux1/2 -> [vq]  "vq"
  [wt] -> Current abc to dq0/2
  Rate Transition/1 -> PLL (3ph)/1
  PLL (3ph)/1 -> Gain2/1
  [Vabcpu] -> Rate Transition/1
  Gain2/1 -> [we]
  PWM Generator (2-Level)/1 -> Vref/1
  Constant/1 -> Sum3/2
  Sum3/1 -> [wt]
  Gain3/1 -> Sum3/1
  Sawtooth Generator/1 -> Gain3/1
  PI Controller q/1 -> Sum5/1
  PI Controller d/1 -> Sum4/1
  [vq_cont] -> Mux1/2
  dq0 to abc/1 -> Saturation/1  "Vabc_ref"
  Mux1/1 -> dq0 to abc/1
  dq1/1 -> Mux1/3
  [vd_cont] -> Mux1/1
  [wt] -> dq0 to abc/2
  PLL (3ph)/2 -> Terminator2/1
  [we] -> " "/2
  [we] -> " 1"/2
  [vq] -> Sum2/2
  [vd] -> Sum1/2

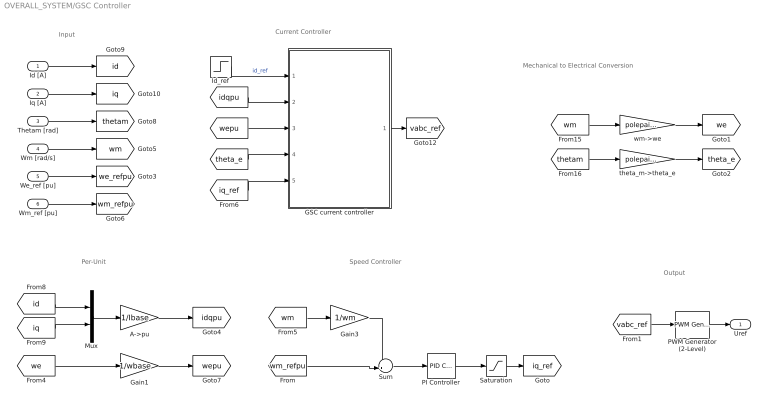
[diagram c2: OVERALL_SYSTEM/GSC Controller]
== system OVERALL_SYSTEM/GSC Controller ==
  note: Input
  note: Speed Controller
  note: Per-Unit
  note: Current Controller
  note: Mechanical to Electrical Conversion
  note: Output
  Id [A] : Inport
  Iq [A] : Inport  Port=2
  Thetam [rad] : Inport  Port=3
  Wm [rad/s] : Inport  Port=4
  We_ref [pu] : Inport  Port=5
  Wm_ref [pu] : Inport  Port=6
  A->pu : Gain  Gain=1/Ibase
  GSC current controller : Subsystem
  Gain1 : Gain  Gain=1/wbase
  Gain3 : Gain  Gain=1/wm
  Id_ref : Step  Time=0  After=0  SampleTime=0
  Mux : Mux  Inputs=2
  PI Controller : simulink/Continuous/PID Controller  Controller=PI  TimeDomain=Continuous-time  SampleTime=-1  IntegratorMethod=Forward Euler  FilterMethod=Forward Euler  Form=Parallel  UseFilter=on  ControllerParametersSource=internal  P=Kpw+3  I=Kiw+3  D=10  N=100  InitialConditionSource=internal  InitialConditionForIntegrator=0  InitialConditionForFilter=0  ExternalReset=none  LimitOutput=off  UpperSaturationLimit=inf  LowerSaturationLimit=-inf  LinearizeAsGain=on  AntiWindupMode=none  Kb=1  TrackingMode=off  Kt=1  PParamMin=[]  PParamMax=[]  IParamMin=[]  IParamMax=[]  DParamMin=[]  DParamMax=[]  NParamMin=[]  NParamMax=[]  KbParamMin=[]  KbParamMax=[]  KtParamMin=[]  KtParamMax=[]  POutMin=[]  POutMax=[]  IOutMin=[]  IOutMax=[]  DOutMin=[]  DOutMax=[]  NOutMin=[]  NOutMax=[]  KbOutMin=[]  KbOutMax=[]  KtOutMin=[]  KtOutMax=[]  IntegratorOutMin=[]  IntegratorOutMax=[]  FilterOutMin=[]  FilterOutMax=[]  SumOutMin=[]  SumOutMax=[]  SumI1OutMin=[]  SumI1OutMax=[]  SumI2OutMin=[]  SumI2OutMax=[]  SumI3OutMin=[]  SumI3OutMax=[]  SumDOutMin=[]  SumDOutMax=[]  SaturationOutMin=[]  SaturationOutMax=[]  IntegratorContinuousStateAttributes=''  IntegratorStateMustResolveToSignalObject=off  IntegratorRTWStateStorageClass=Auto  FilterContinuousStateAttributes=''  FilterStateMustResolveToSignalObject=off  FilterRTWStateStorageClass=Auto  DifferentiatorICPrevScaledInput=0  DifferentiatorOutMin=[]  DifferentiatorOutMax=[]
  PWM Generator (2-Level) : powerlib_meascontrol/Pulse & Signal Generators/PWM Generator (2-Level)  ModulatorType=Three-phase bridge (6 pulses)  ModulatorMode=Unsynchronized  Fc=fsw  Pc=90  nF=27  MinMax="[ -1  1 ]"  SamplingTechnique=Natural  ModulatingSignals=off  m=0.8  Freq=60  Phase=0  Ts=0  ShowCarrierOutport=off
  Saturation : Saturate  UpperLimit=1  LowerLimit=-2
  Sum : Sum  Inputs=-+|
  theta_m->theta_e : Gain  Gain=polepairs
  wm->we : Gain  Gain=polepairs
  Uref : Outport
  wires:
  [wepu] -> GSC current controller/3(we [pu])
  [iq_ref] -> GSC current controller/5(iq_ref [pu])
  PI Controller/1 -> Saturation/1
  wm->we/1 -> [we]
  [theta_e] -> GSC current controller/4(wt [rad])
  [iq] -> Mux/2
  [idqpu] -> GSC current controller/2(idq [pu])
  [we] -> Gain1/1
  [id] -> Mux/1
  A->pu/1 -> [idqpu]
  [thetam] -> theta_m->theta_e/1
  Mux/1 -> A->pu/1
  Gain1/1 -> [wepu]
  Saturation/1 -> [iq_ref]
  Sum/1 -> PI Controller/1
  [wm] -> wm->we/1
  [wm] -> Gain3/1
  theta_m->theta_e/1 -> [theta_e]
  Id_ref/1 -> GSC current controller/1("id_ref [pu] ")  "id_ref"
  GSC current controller/1("Vabc_ref [pu] ") -> [vabc_ref]
  Wm [rad/s]/1 -> [wm]
  Thetam [rad]/1 -> [thetam]
  Id [A]/1 -> [id]
  Iq [A]/1 -> [iq]
  We_ref [pu]/1 -> [we_refpu]
  Gain3/1 -> Sum/1
  Wm_ref [pu]/1 -> [wm_refpu]
  PWM Generator (2-Level)/1 -> Uref/1
  [wm_refpu] -> Sum/2
  [vabc_ref] -> PWM Generator (2-Level)/1

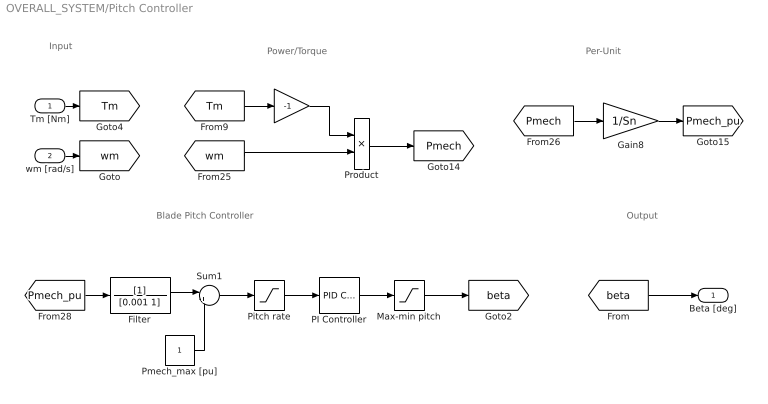
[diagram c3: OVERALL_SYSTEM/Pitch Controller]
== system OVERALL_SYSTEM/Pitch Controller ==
  note: Blade Pitch Controller
  note: Power/Torque
  note: Input
  note: Per-Unit
  note: Output
  Tm [Nm] : Inport
  wm [rad/s] : Inport  Port=2
  " " : Gain  Gain=-1
  Filter : TransferFcn  Denominator=[0.001 1]
  Gain8 : Gain  Gain=1/Sn
  Max-min pitch : Saturate  UpperLimit=beta_max  LowerLimit=beta_min  SampleTime=Ts
  PI Controller : simulink/Continuous/PID Controller  Controller=PI  TimeDomain=Continuous-time  SampleTime=-1  IntegratorMethod=Forward Euler  FilterMethod=Forward Euler  Form=Parallel  UseFilter=on  ControllerParametersSource=internal  P=Kpb  I=Kib  D=10  N=100  InitialConditionSource=internal  InitialConditionForIntegrator=0  InitialConditionForFilter=0  ExternalReset=none  LimitOutput=off  UpperSaturationLimit=inf  LowerSaturationLimit=-inf  LinearizeAsGain=on  AntiWindupMode=none  Kb=1  TrackingMode=off  Kt=1  PParamMin=[]  PParamMax=[]  IParamMin=[]  IParamMax=[]  DParamMin=[]  DParamMax=[]  NParamMin=[]  NParamMax=[]  KbParamMin=[]  KbParamMax=[]  KtParamMin=[]  KtParamMax=[]  POutMin=[]  POutMax=[]  IOutMin=[]  IOutMax=[]  DOutMin=[]  DOutMax=[]  NOutMin=[]  NOutMax=[]  KbOutMin=[]  KbOutMax=[]  KtOutMin=[]  KtOutMax=[]  IntegratorOutMin=[]  IntegratorOutMax=[]  FilterOutMin=[]  FilterOutMax=[]  SumOutMin=[]  SumOutMax=[]  SumI1OutMin=[]  SumI1OutMax=[]  SumI2OutMin=[]  SumI2OutMax=[]  SumI3OutMin=[]  SumI3OutMax=[]  SumDOutMin=[]  SumDOutMax=[]  SaturationOutMin=[]  SaturationOutMax=[]  IntegratorContinuousStateAttributes=''  IntegratorStateMustResolveToSignalObject=off  IntegratorRTWStateStorageClass=Auto  FilterContinuousStateAttributes=''  FilterStateMustResolveToSignalObject=off  FilterRTWStateStorageClass=Auto  DifferentiatorICPrevScaledInput=0  DifferentiatorOutMin=[]  DifferentiatorOutMax=[]
  Pitch rate : Saturate  UpperLimit=beta_r  LowerLimit=0  SampleTime=Ts
  Pmech_max [pu] : Constant
  Product : Product
  Sum1 : Sum  Inputs=|+-
  Beta [deg] : Outport
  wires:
  Max-min pitch/1 -> [beta]
  " "/1 -> Product/1
  [wm] -> Product/2
  Pmech_max [pu]/1 -> Sum1/2
  [Tm] -> " "/1
  Pitch rate/1 -> PI Controller/1
  PI Controller/1 -> Max-min pitch/1
  [Pmech] -> Gain8/1
  Product/1 -> [Pmech]
  Tm [Nm]/1 -> [Tm]
  Gain8/1 -> [Pmech_pu]
  wm [rad/s]/1 -> [wm]
  [beta] -> Beta [deg]/1
  Filter/1 -> Sum1/1
  Sum1/1 -> Pitch rate/1
  [Pmech_pu] -> Filter/1

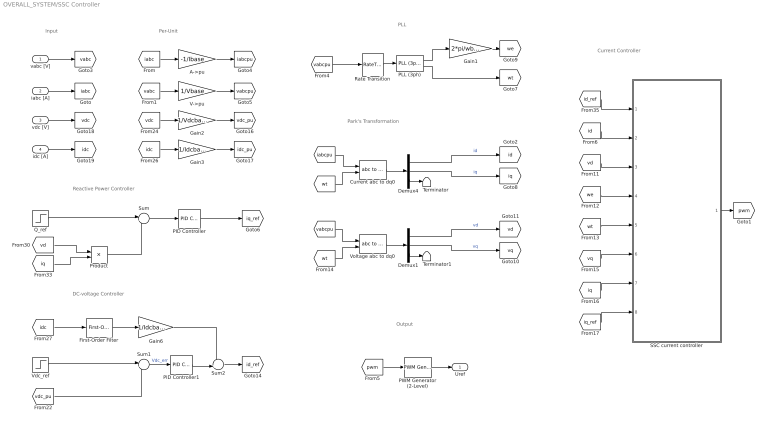
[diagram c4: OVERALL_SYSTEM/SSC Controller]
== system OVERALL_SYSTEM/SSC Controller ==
  note: Output
  note: Input
  note: Reactive Power Controller
  note: Park's Transformation
  note: PLL
  note: Per-Unit
  note: DC-voltage Controller
  note: Current Controller
  vabc [V] : Inport
  iabc [A] : Inport  Port=2
  vdc [V] : Inport  Port=3
  idc [A] : Inport  Port=4
  A->pu : Gain  Gain=-1/Ibase
  Current abc to dq0 : powerlib_meascontrol/Transformations/abc to dq0  Alignment=90 degrees behind phase A axis
  Demux1 : Demux  Outputs=3
  Demux4 : Demux  Outputs=3
  First-Order Filter : powerlib_meascontrol/Filters/First-Order Filter  FilterType=Lowpass  Tc=1.5e-3  Ts=0  Initialize=on  Vac_Init=[0, 0, 0]  Vdc_Init=Idcbase  PlotResponse=off  FreqRange="[0,  200,  1]"
  Gain1 : Gain  Gain=2*pi/wbase
  Gain2 : Gain  Gain=1/Vdcbase
  Gain3 : Gain  Gain=1/Idcbase
  Gain6 : Gain  Gain=1/Idcbase
  PID Controller : simulink/Continuous/PID Controller  Controller=PI  TimeDomain=Continuous-time  SampleTime=-1  IntegratorMethod=Forward Euler  FilterMethod=Forward Euler  Form=Parallel  UseFilter=on  ControllerParametersSource=internal  P=Kpq  I=Kiq  D=0  N=100  InitialConditionSource=internal  InitialConditionForIntegrator=0  InitialConditionForFilter=0  ExternalReset=none  LimitOutput=off  UpperSaturationLimit=inf  LowerSaturationLimit=-inf  LinearizeAsGain=on  AntiWindupMode=none  Kb=1  TrackingMode=off  Kt=1  PParamMin=[]  PParamMax=[]  IParamMin=[]  IParamMax=[]  DParamMin=[]  DParamMax=[]  NParamMin=[]  NParamMax=[]  KbParamMin=[]  KbParamMax=[]  KtParamMin=[]  KtParamMax=[]  POutMin=[]  POutMax=[]  IOutMin=[]  IOutMax=[]  DOutMin=[]  DOutMax=[]  NOutMin=[]  NOutMax=[]  KbOutMin=[]  KbOutMax=[]  KtOutMin=[]  KtOutMax=[]  IntegratorOutMin=[]  IntegratorOutMax=[]  FilterOutMin=[]  FilterOutMax=[]  SumOutMin=[]  SumOutMax=[]  SumI1OutMin=[]  SumI1OutMax=[]  SumI2OutMin=[]  SumI2OutMax=[]  SumI3OutMin=[]  SumI3OutMax=[]  SumDOutMin=[]  SumDOutMax=[]  SaturationOutMin=[]  SaturationOutMax=[]  IntegratorContinuousStateAttributes=''  IntegratorStateMustResolveToSignalObject=off  IntegratorRTWStateStorageClass=Auto  FilterContinuousStateAttributes=''  FilterStateMustResolveToSignalObject=off  FilterRTWStateStorageClass=Auto  DifferentiatorICPrevScaledInput=0  DifferentiatorOutMin=[]  DifferentiatorOutMax=[]
  PID Controller1 : simulink/Continuous/PID Controller  Controller=PI  TimeDomain=Continuous-time  SampleTime=-1  IntegratorMethod=Forward Euler  FilterMethod=Forward Euler  Form=Parallel  UseFilter=on  ControllerParametersSource=internal  P=-(Kpdc)  I=-(Kidc)  D=0  N=100  InitialConditionSource=internal  InitialConditionForIntegrator=0  InitialConditionForFilter=0  ExternalReset=none  LimitOutput=off  UpperSaturationLimit=inf  LowerSaturationLimit=-inf  LinearizeAsGain=on  AntiWindupMode=none  Kb=1  TrackingMode=off  Kt=1  PParamMin=[]  PParamMax=[]  IParamMin=[]  IParamMax=[]  DParamMin=[]  DParamMax=[]  NParamMin=[]  NParamMax=[]  KbParamMin=[]  KbParamMax=[]  KtParamMin=[]  KtParamMax=[]  POutMin=[]  POutMax=[]  IOutMin=[]  IOutMax=[]  DOutMin=[]  DOutMax=[]  NOutMin=[]  NOutMax=[]  KbOutMin=[]  KbOutMax=[]  KtOutMin=[]  KtOutMax=[]  IntegratorOutMin=[]  IntegratorOutMax=[]  FilterOutMin=[]  FilterOutMax=[]  SumOutMin=[]  SumOutMax=[]  SumI1OutMin=[]  SumI1OutMax=[]  SumI2OutMin=[]  SumI2OutMax=[]  SumI3OutMin=[]  SumI3OutMax=[]  SumDOutMin=[]  SumDOutMax=[]  SaturationOutMin=[]  SaturationOutMax=[]  IntegratorContinuousStateAttributes=''  IntegratorStateMustResolveToSignalObject=off  IntegratorRTWStateStorageClass=Auto  FilterContinuousStateAttributes=''  FilterStateMustResolveToSignalObject=off  FilterRTWStateStorageClass=Auto  DifferentiatorICPrevScaledInput=0  DifferentiatorOutMin=[]  DifferentiatorOutMax=[]
  PLL (3ph) : powerlib_meascontrol/PLL/PLL (3ph)  Fmin=35  Par_Init=[0, 50]  ParK=[180, 3200, 1]  TcD=1e-4  MaxRateChangeFreq=12  FilterCutOffFreq=25  Ts=0  AGC=on
  PWM Generator (2-Level) : powerlib_meascontrol/Pulse & Signal Generators/PWM Generator (2-Level)  ModulatorType=Three-phase bridge (6 pulses)  ModulatorMode=Unsynchronized  Fc=fsw  Pc=90  nF=27  MinMax="[ -1  1 ]"  SamplingTechnique=Natural  ModulatingSignals=off  m=0.8  Freq=60  Phase=0  Ts=0  ShowCarrierOutport=off
  Product : Product
  Q_ref : Step  Time=0  After=0  SampleTime=0
  Rate Transition : RateTransition  OutPortSampleTime=Ts
  SSC current controller : Subsystem
  Sum : Sum  Inputs=|+-
  Sum1 : Sum  Inputs=|+-
  Sum2 : Sum  Inputs=-+|
  Terminator : Terminator
  Terminator1 : Terminator
  V->pu : Gain  Gain=1/Vbase
  Vdc_ref : Step  Time=0  Before=1  SampleTime=40
  Voltage abc to dq0 : powerlib_meascontrol/Transformations/abc to dq0  Alignment=90 degrees behind phase A axis
  Uref : Outport
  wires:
  [wt] -> Voltage abc to dq0/2
  PLL (3ph)/2 -> [wt]
  Q_ref/1 -> Sum/1
  Demux1/3 -> Terminator1/1
  A->pu/1 -> [iabcpu]
  Gain3/1 -> [idc_pu]
  [iabc] -> A->pu/1
  [iq_ref] -> SSC current controller/8(iq_ref [pu])
  [vd] -> SSC current controller/3(vd [pu])
  Rate Transition/1 -> PLL (3ph)/1
  Demux4/1 -> [id]  "id"
  PLL (3ph)/1 -> Gain1/1
  [vabc] -> V->pu/1
  [we] -> SSC current controller/4(we [rad/s])
  [vabcpu] -> Rate Transition/1
  [id] -> SSC current controller/2(id [pu])
  [idc] -> Gain3/1
  Demux4/3 -> Terminator/1
  Sum1/1 -> PID Controller1/1  "Vdc_err"
  [vabcpu] -> Voltage abc to dq0/1
  Demux4/2 -> [iq]  "iq"
  Current abc to dq0/1 -> Demux4/1
  Voltage abc to dq0/1 -> Demux1/1
  SSC current controller/1("Vabc_ref [pu] ") -> [pwm]
  [id_ref] -> SSC current controller/1("id_ref [pu] ")
  Vdc_ref/1 -> Sum1/1
  [vdc_pu] -> Sum1/2
  [vq] -> SSC current controller/6(vq [pu])
  Gain2/1 -> [vdc_pu]
  Sum/1 -> PID Controller/1
  [iq] -> SSC current controller/7(iq [pu])
  Gain1/1 -> [we]
  [vdc] -> Gain2/1
  Demux1/1 -> [vd]  "vd"
  V->pu/1 -> [vabcpu]
  [iabcpu] -> Current abc to dq0/1
  Demux1/2 -> [vq]  "vq"
  [wt] -> SSC current controller/5(wt [rad])
  [wt] -> Current abc to dq0/2
  vabc [V]/1 -> [vabc]
  iabc [A]/1 -> [iabc]
  vdc [V]/1 -> [vdc]
  idc [A]/1 -> [idc]
  [pwm] -> PWM Generator (2-Level)/1
  PWM Generator (2-Level)/1 -> Uref/1
  PID Controller/1 -> [iq_ref]
  PID Controller1/1 -> Sum2/2
  [idc] -> First-Order Filter/1
  First-Order Filter/1 -> Gain6/1
  Gain6/1 -> Sum2/1
  Sum2/1 -> [id_ref]
  [vd] -> Product/1
  [iq] -> Product/2
  Product/1 -> Sum/2

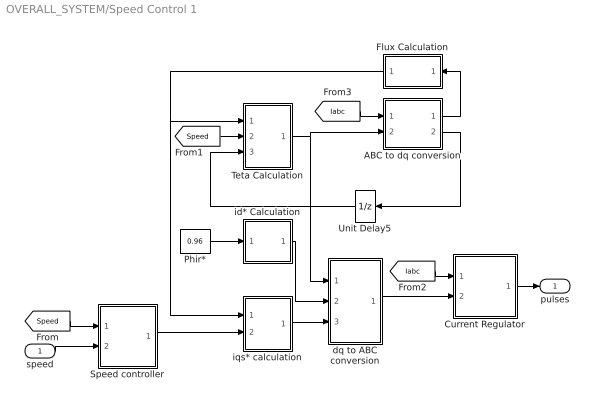
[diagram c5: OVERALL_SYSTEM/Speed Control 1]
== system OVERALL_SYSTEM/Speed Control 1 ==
  speed : Inport
  ABC to dq conversion : Subsystem
  Current Regulator : Subsystem
  Flux Calculation : Subsystem
  Phir* : Constant  Value=0.96
  Speed controller : Subsystem
  Teta Calculation : Subsystem
  Unit Delay5 : UnitDelay  SampleTime=Ts
  dq to ABC conversion : Subsystem
  id* Calculation : Subsystem
  iqs* calculation : Subsystem
  pulses : Outport
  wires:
  dq to ABC conversion/1(Iabc*) -> Current Regulator/2(Iabc*)
  Speed controller/1(Te*) -> iqs* calculation/2(Te*)
  Phir*/1 -> id* Calculation/1(Phir*)
  ABC to dq conversion/1(Id) -> Flux Calculation/1(Id)
  id* Calculation/1(Id*) -> dq to ABC conversion/2(Id*)
  Flux Calculation/1(Phir) -> Teta Calculation/1(Phir), iqs* calculation/1(Phir)
  ABC to dq conversion/2(Iq) -> Unit Delay5/1
  Unit Delay5/1 -> Teta Calculation/3(Iq)
  iqs* calculation/1(Iq*) -> dq to ABC conversion/3(Iq*)
  Teta Calculation/1(Teta) -> dq to ABC conversion/1(Teta), ABC to dq conversion/2(Teta)
  [Speed] -> Speed controller/1(w)
  [Speed] -> Teta Calculation/2(wm)
  [Iabc] -> Current Regulator/1(Iabc)
  [Iabc] -> ABC to dq conversion/1(Iabc)
  speed/1 -> Speed controller/2(w*)
  Current Regulator/1(Pulses) -> pulses/1

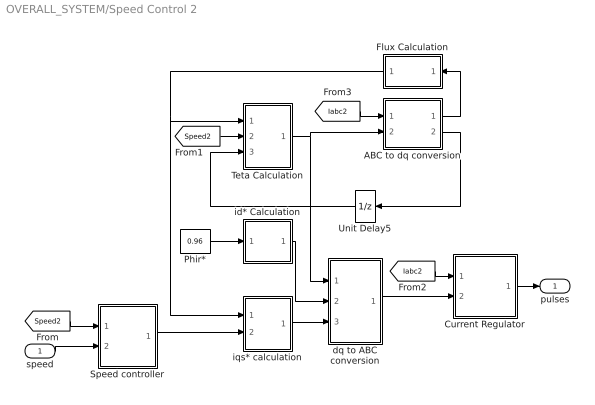
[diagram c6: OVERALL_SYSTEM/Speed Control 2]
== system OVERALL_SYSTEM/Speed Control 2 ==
  speed : Inport
  ABC to dq conversion : Subsystem
  Current Regulator : Subsystem
  Flux Calculation : Subsystem
  Phir* : Constant  Value=0.96
  Speed controller : Subsystem
  Teta Calculation : Subsystem
  Unit Delay5 : UnitDelay  SampleTime=Ts
  dq to ABC conversion : Subsystem
  id* Calculation : Subsystem
  iqs* calculation : Subsystem
  pulses : Outport
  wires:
  dq to ABC conversion/1(Iabc*) -> Current Regulator/2(Iabc*)
  Speed controller/1(Te*) -> iqs* calculation/2(Te*)
  Phir*/1 -> id* Calculation/1(Phir*)
  ABC to dq conversion/1(Id) -> Flux Calculation/1(Id)
  id* Calculation/1(Id*) -> dq to ABC conversion/2(Id*)
  Flux Calculation/1(Phir) -> Teta Calculation/1(Phir), iqs* calculation/1(Phir)
  ABC to dq conversion/2(Iq) -> Unit Delay5/1
  Unit Delay5/1 -> Teta Calculation/3(Iq)
  iqs* calculation/1(Iq*) -> dq to ABC conversion/3(Iq*)
  Teta Calculation/1(Teta) -> dq to ABC conversion/1(Teta), ABC to dq conversion/2(Teta)
  [Speed2] -> Speed controller/1(w)
  [Speed2] -> Teta Calculation/2(wm)
  [Iabc2] -> Current Regulator/1(Iabc)
  [Iabc2] -> ABC to dq conversion/1(Iabc)
  speed/1 -> Speed controller/2(w*)
  Current Regulator/1(Pulses) -> pulses/1

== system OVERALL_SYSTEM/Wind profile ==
  Demux : Demux  Tag=STV Demux  Outputs=1
  FromWs : FromWorkspace  Tag=STV FromWs  VariableName=tuvar  SampleTime=0
  Final Wind : Outport  Tag=STV Outport
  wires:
  FromWs/1 -> Demux/1
  Demux/1 -> Final Wind/1

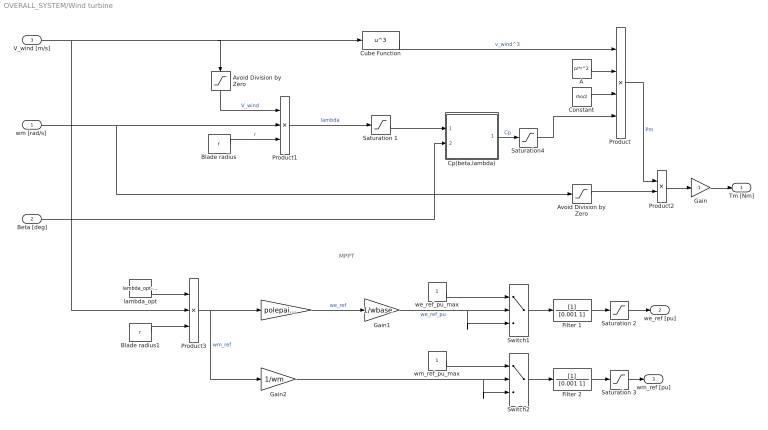
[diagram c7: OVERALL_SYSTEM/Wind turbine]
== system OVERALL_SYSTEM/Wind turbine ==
  note: MPPT
  "wm [rad/s] " : Inport
  Beta [deg] : Inport  Port=2
  V_wind [m/s] : Inport  Port=3
  " " : Gain  Gain=polepairs
  A : Constant  Value=pi*r^2
  Avoid Division by Zero : Saturate  UpperLimit=1e6  LowerLimit=1e-6
  "Avoid Division by Zero " : Saturate  UpperLimit=1e6  LowerLimit=1e-6
  Blade radius : Constant  Value=r
  Blade radius1 : Constant  Value=r
  Constant : Constant  Value=rho/2
  Cp(beta,lambda) : Subsystem
  Cube Function : Fcn  Expr=u^3
  Filter 1 : TransferFcn  Denominator=[0.001 1]
  Filter 2 : TransferFcn  Denominator=[0.001 1]
  Gain : Gain  Gain=-1
  Gain1 : Gain  Gain=1/wbase
  Gain2 : Gain  Gain=1/wm
  "Product " : Product  Inputs=4
  Product1 : Product  Inputs=/**
  Product2 : Product  Inputs=*/
  Product3 : Product  Inputs=**/
  Saturation 1 : Saturate  UpperLimit=inf  LowerLimit=1e-6
  Saturation 2 : Saturate  UpperLimit=1  LowerLimit=-1
  Saturation 3 : Saturate  UpperLimit=1  LowerLimit=-1
  Saturation4 : Saturate  UpperLimit=Cp_max  LowerLimit=1e-6
  Switch1 : Switch  Threshold=1.1
  Switch2 : Switch  Threshold=1.1
  lambda_opt : Constant  Value=lambda_opt-0.0386
  we_ref_pu_max : Constant
  wm_ref_pu_max : Constant
  Tm [Nm] : Outport
  we_ref [pu] : Outport  Port=2
  wm_ref [pu] : Outport  Port=3
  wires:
  Beta [deg]/1 -> Cp(beta,lambda)/2(beta)
  V_wind [m/s]/1 -> "Avoid Division by Zero "/1, Cube Function/1, Product3/2
  Product2/1 -> Gain/1
  Avoid Division by Zero/1 -> Product2/2
  "Product "/1 -> Product2/1  "Pm"
  Saturation 1/1 -> Cp(beta,lambda)/1(lambda)
  Product1/1 -> Saturation 1/1  "lambda"
  "wm [rad/s] "/1 -> Product1/2, Avoid Division by Zero/1
  A/1 -> "Product "/2
  Blade radius/1 -> Product1/3  "r"
  Cp(beta,lambda)/1(Cp) -> Saturation4/1  "Cp"
  Cube Function/1 -> "Product "/1  "v_wind^3"
  Constant/1 -> "Product "/3
  "Avoid Division by Zero "/1 -> Product1/1  "V_wind"
  Blade radius1/1 -> Product3/3
  lambda_opt/1 -> Product3/1
  Product3/1 -> Gain2/1, " "/1  "wm_ref"
  " "/1 -> Gain1/1  "we_ref"
  Gain1/1 -> Switch1/3, Switch1/2  "we_ref_pu"
  Saturation 2/1 -> we_ref [pu]/1
  we_ref_pu_max/1 -> Switch1/1
  Switch1/1 -> Filter 1/1
  Saturation 3/1 -> wm_ref [pu]/1
  Gain2/1 -> Switch2/3, Switch2/2
  Filter 2/1 -> Saturation 3/1
  Gain/1 -> Tm [Nm]/1
  Saturation4/1 -> "Product "/4
  wm_ref_pu_max/1 -> Switch2/1
  Switch2/1 -> Filter 2/1
  Filter 1/1 -> Saturation 2/1
